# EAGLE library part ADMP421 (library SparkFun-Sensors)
Omnidirectional bottom-port MEMS microphone (digital output)
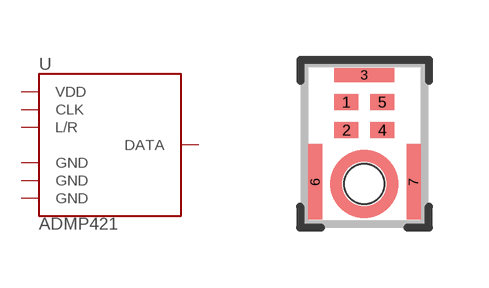
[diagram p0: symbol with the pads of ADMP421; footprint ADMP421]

Designator prefix -

## ADMP421  [ADMP421]
1  CLK
2  L/R
3  GND
4  VDD
5  DATA
6  GND
7  GND

## Footprint ADMP421 (pad centres in mm)
smd 0.6 x 0.4: 1 -0.45,2.05; 2 -0.45,1.35; 4 0.45,1.35; 5 0.45,2.05
smd 1.5 x 0.35: 3 0,2.73
smd 0.35 x 1.9: 6 -1.23,0.06; 7 1.23,0.06
hole 1 at 0,0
